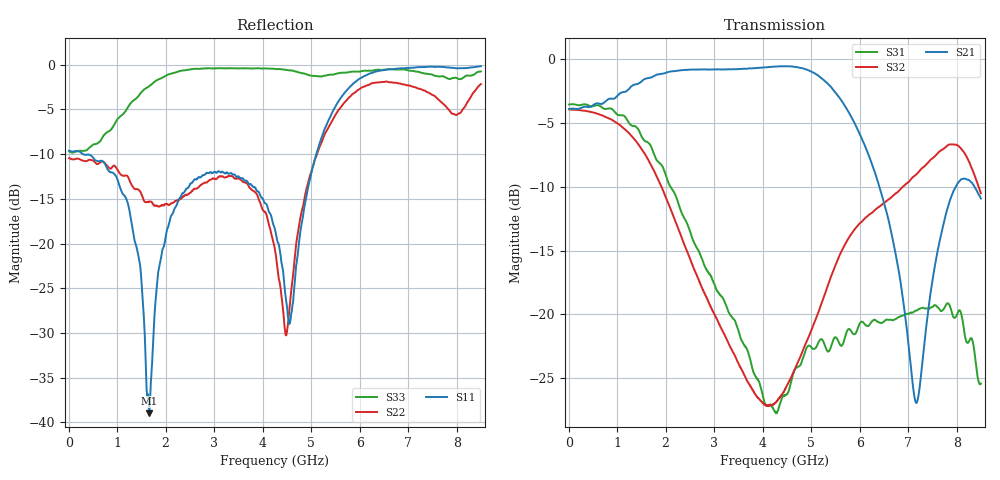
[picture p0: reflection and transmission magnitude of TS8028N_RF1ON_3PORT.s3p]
!Created with skrf (http://scikit-rf.org).
# GHz S RI R 50.0
!freq ReS11 ImS11 ReS12 ImS12 ReS13 ImS13
! ReS21 ImS21 ReS22 ImS22 ReS23 ImS23
! ReS31 ImS31 ReS32 ImS32 ReS33 ImS33
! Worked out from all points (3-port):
!   1601 points, 10 MHz to 8.5 GHz, reference 50 ohm
!   strongest paths, dB at 10 MHz, 2.132 GHz, 4.255 GHz, 6.378 GHz, 8.5 GHz:
!     S21: -3.9, -0.9, -0.6, -9.6, -10.9
!     S32: -3.9, -12.0, -26.9, -11.6, -10.5
!     S31: -3.5, -10.2, -27.6, -20.6, -25.4
!   lowest |S11| = -39.0 dB at 1.66 GHz (marker M1), VSWR 1.02, Z = 49.2 - j0.821 ohm
!   |S11| at or under -10 dB: 294.9 MHz to 5.106 GHz (4.811 GHz wide, 178 % of centre)
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0.01  -0.3308 0.00661  0.6384 0.00189  0.6654 -0.0038
      0.6381 0.0018  -0.3002 0.00737  0.6364 -0.00566
      0.6651 -0.00389  0.6365 -0.00552  -0.3273 0.013
1.203906  -0.1476 0.0902  0.7348 -0.1628  0.1746 -0.5534
          0.7349 -0.1629  -0.1844 0.153  0.1003 -0.5129
          0.1747 -0.5538  0.1005 -0.5133  0.4873 0.2918
1.660244  -0.00752 -0.00833  0.7692 -0.3503  -0.0828 -0.4602
          0.7688 -0.3505  -0.1401 0.0985  -0.1454 -0.3697
          -0.0824 -0.46  -0.1452 -0.3695  0.7368 -0.1786
2.360669  0.1034 -0.1612  0.6401 -0.6443  -0.1736 -0.1695
          0.6399 -0.6443  -0.1476 0.1082  -0.1668 -0.0979
          -0.1739 -0.1695  -0.1667 -0.0976  0.5407 -0.7554
4.255  -0.0621 -0.1025  -0.1865 -0.9183  -0.0363 -0.0199
       -0.1874 -0.9179  -0.0146 0.0909  -0.00586 0.0447
       -0.0365 -0.0198  -0.00582 0.0446  -0.5868 -0.7452
5.263187  0.1848 0.3844  -0.7148 -0.4189  -0.0188 0.0751
          -0.7149 -0.4185  -0.3965 0.0497  0.1047 0.0531
          -0.0187 0.0751  0.1046 0.0529  0.00495 0.8677
6.515462  0.8491 0.3974  -0.2386 0.1236  0.0484 -0.0813
          -0.2377 0.124  0.035 0.8025  0.1808 -0.2059
          0.0481 -0.0812  0.1819 -0.206  0.9322 -0.112
7.428138  0.9254 0.3104  -0.0275 -0.1052  -0.0278 -0.1017
          -0.0277 -0.105  0.6945 0.0665  -0.0502 -0.3934
          -0.028 -0.1014  -0.0494 -0.3942  0.8501 -0.2549
7.958762  0.891 0.3576  -0.2076 -0.2301  -0.0797 -0.0546
          -0.209 -0.2297  -0.0546 -0.5247  -0.3773 -0.27
          -0.0801 -0.0548  -0.3756 -0.2719  0.8226 -0.1965
8.5  0.8758 0.4453  -0.2839 0.0115  -0.0518 0.0131
     -0.2843 0.0121  -0.6107 0.4852  -0.283 0.0964
     -0.0519 0.0131  -0.2828 0.0953  0.9011 -0.1754
